(* Logix 5000 AddOnInstructionDefinition export CM1T_CMLDataExchange; software revision 20.00 *)

TYPE CM1T_CMLDriveStatus :
STRUCT
   StatusValue : SINT;   // Indicates status and error type
   StatusValue1 : SINT;   // Additional status values
   In_Position : BOOL;   // Drive is in position and ready to move
   Moving : BOOL;   // Drive is currently moving
   Disabled : BOOL;   // Drive is disabled
   Error : BOOL;   // Drive is in an error state
   HomeAchieved : BOOL;   // Home achieved
END_STRUCT
END_TYPE

TYPE CM1T_CMLAxis :   // CML Axis
STRUCT
   Input : SINT[60];   // Data coming from the CM1-T
   Output : SINT[44];   // Data going to the CM1-T
   us50Counter : DINT;   // Controller 50us counter
   DriveStatus : CM1T_CMLDriveStatus;   // Shows status of the drive
   PositionActual : DINT;   // Actual position of the drive
   TargetActual : DINT;   // 1ms position target
   PositionError : DINT;   // Error between the current drive position and the instantaneous target position
   SpeedActual : DINT;   // Actual speed of the drive
   CurrentActual : INT;   // 0.1% of rated current
   OverloadActual : INT;   // 0.1% of overload torque
   DCVoltage : INT;   // DC voltage bus. 0.1V unit
   AnalogIN : INT;   // Value of 10bit analog input
   DigitalIN : SINT;   // Read the digital inputs
   DigitalOUT : SINT;   // Set the digital outputs
   Temperature : SINT;   // Temperature of the drive
   ErrorCode : SINT;   // Indicates error in Ethernet/IP module
   WriteValue : DINT[5];   // Write value array
   ReadValue : DINT[5];   // Read Value array
   WriteAddr : INT[5];   // Write Address array
   ReadAddr : INT[5];   // Read Address array
   ReadValueAddr : INT[5];   // Address of ReadValue
END_STRUCT
END_TYPE

ADD_ON_INSTRUCTION CM1T_CMLDataExchange   (* revision 1.2, vendor Myostat Motion Control *)
// CM1T CML Data Exchange
VAR_IN_OUT
   DriveInput : AB:ETHERNET_MODULE_SINT_60Bytes:I:0; {required}
   DriveOutput : AB:ETHERNET_MODULE_SINT_44Bytes:O:0; {required}
        .DATA[0]   // Copy outputs to drive
   CM1T_CMLAxis : CM1T_CMLAxis; {required}
        .CONTROLWORD.START   // Controlword.Start Off
        .INPUT   // Copy input from drive
        .OUTPUT[0]   // Write Value1
        .OUTPUT[4]   // Write Value2
        .OUTPUT[8]   // Write Value3
        .OUTPUT[10]   // AccelerationTarget
        .OUTPUT[12]   // Write Value4
        .OUTPUT[14]   // Controlword
        .OUTPUT[16]   // Write Value5
        .OUTPUT[17]   // WriteData
        .OUTPUT[18]   // WriteAddress
        .OUTPUT[20]   // Write Addr1
        .OUTPUT[21]   // Digital OUT
        .OUTPUT[22]   // Write Addr2
        .OUTPUT[24]   // Write Addr3
        .OUTPUT[26]   // Write Addr4
        .OUTPUT[28]   // Write Addr5
        .OUTPUT[30]   // Read Addr1
        .OUTPUT[32]   // Read Addr2
        .OUTPUT[34]   // Read Addr3
        .OUTPUT[36]   // Read Addr4
        .OUTPUT[38]   // Read Addr5
        .DRIVESTATUS.STATUSVALUE   // Status
        .DRIVESTATUS.IN_POSITION   // In Position
        .DRIVESTATUS.MOVING   // Moving
        .DRIVESTATUS.ERROR   // Error
        .POSITIONACTUAL   // Position
        .POSITIONERROR   // Position Error
        .CURRENTACTUAL   // Current
        .DCVOLTAGE   // DC Voltage
        .ANALOGIN   // AnalogIN
        .DIGITALIN   // DigitalIN
        .MODEOFOPERATIONDISPLAY   // Mode Display
        .SPEEDACTUAL   // Speed
        .OVERLOADACTUAL   // Torque
        .TEMPERATURE   // Temperature
        .ERRORCODE   // ErrorCode
END_VAR

ROUTINE Logic   (* ladder *)
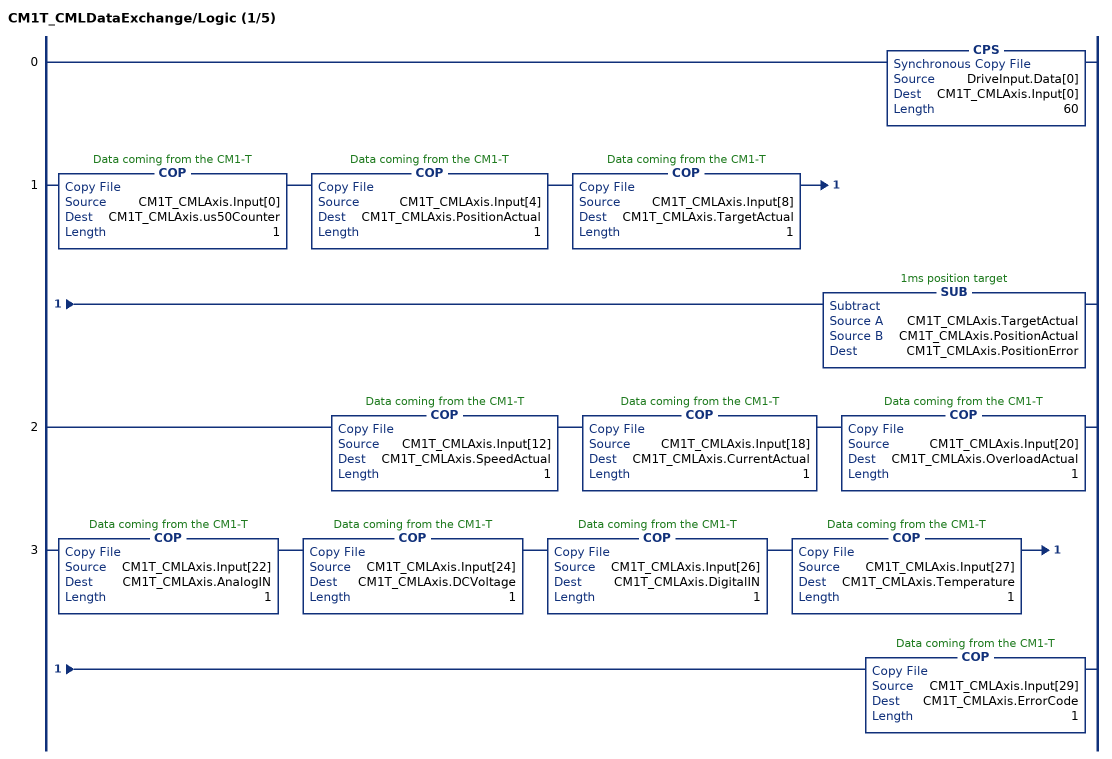
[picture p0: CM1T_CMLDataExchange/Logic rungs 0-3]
   0: CPS(DriveInput.Data[0],CM1T_CMLAxis.Input[0],60);
   1: COP(CM1T_CMLAxis.Input[0],CM1T_CMLAxis.us50Counter,1)COP(CM1T_CMLAxis.Input[4],CM1T_CMLAxis.PositionActual,1)COP(CM1T_CMLAxis.Input[8],CM1T_CMLAxis.TargetActual,1)SUB(CM1T_CMLAxis.TargetActual,CM1T_CMLAxis.PositionActual,CM1T_CMLAxis.PositionError);
   2: COP(CM1T_CMLAxis.Input[12],CM1T_CMLAxis.SpeedActual,1)COP(CM1T_CMLAxis.Input[18],CM1T_CMLAxis.CurrentActual,1)COP(CM1T_CMLAxis.Input[20],CM1T_CMLAxis.OverloadActual,1);
   3: COP(CM1T_CMLAxis.Input[22],CM1T_CMLAxis.AnalogIN,1)COP(CM1T_CMLAxis.Input[24],CM1T_CMLAxis.DCVoltage,1)COP(CM1T_CMLAxis.Input[26],CM1T_CMLAxis.DigitalIN,1)COP(CM1T_CMLAxis.Input[27],CM1T_CMLAxis.Temperature,1)COP(CM1T_CMLAxis.Input[29],CM1T_CMLAxis.ErrorCode,1);
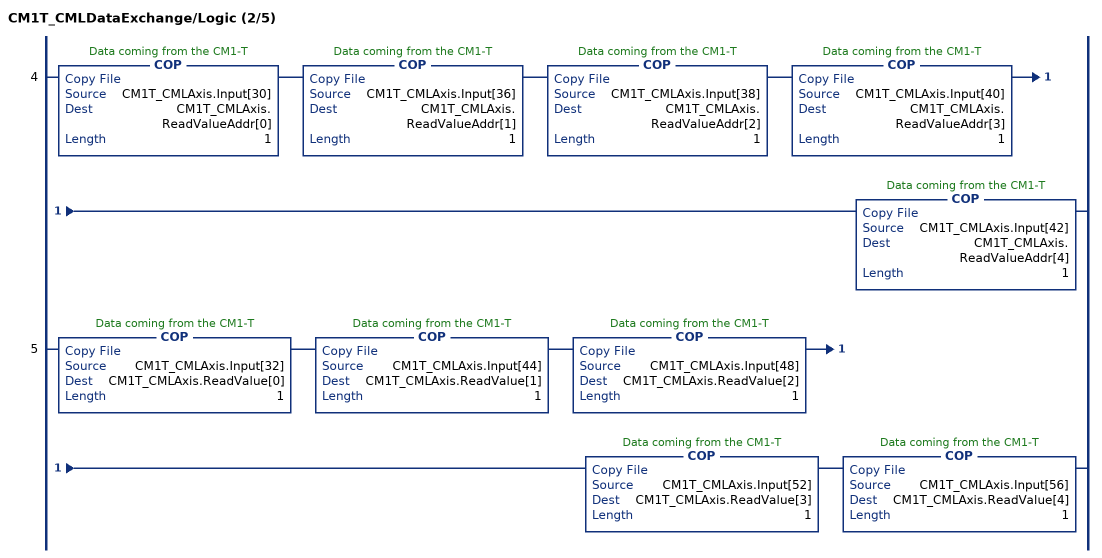
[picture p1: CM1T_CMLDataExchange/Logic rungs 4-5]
   4: COP(CM1T_CMLAxis.Input[30],CM1T_CMLAxis.ReadValueAddr[0],1)COP(CM1T_CMLAxis.Input[36],CM1T_CMLAxis.ReadValueAddr[1],1)COP(CM1T_CMLAxis.Input[38],CM1T_CMLAxis.ReadValueAddr[2],1)COP(CM1T_CMLAxis.Input[40],CM1T_CMLAxis.ReadValueAddr[3],1)COP(CM1T_CMLAxis.Input[42],CM1T_CMLAxis.ReadValueAddr[4],1);
   5: COP(CM1T_CMLAxis.Input[32],CM1T_CMLAxis.ReadValue[0],1)COP(CM1T_CMLAxis.Input[44],CM1T_CMLAxis.ReadValue[1],1)COP(CM1T_CMLAxis.Input[48],CM1T_CMLAxis.ReadValue[2],1)COP(CM1T_CMLAxis.Input[52],CM1T_CMLAxis.ReadValue[3],1)COP(CM1T_CMLAxis.Input[56],CM1T_CMLAxis.ReadValue[4],1);
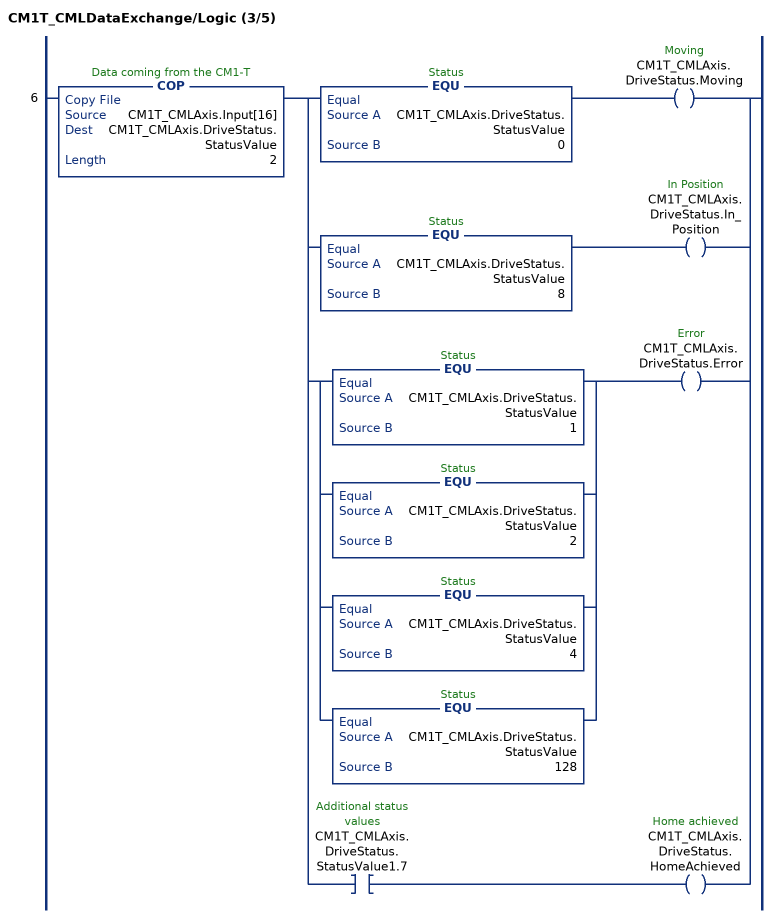
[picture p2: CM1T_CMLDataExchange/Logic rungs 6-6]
   6: COP(CM1T_CMLAxis.Input[16],CM1T_CMLAxis.DriveStatus.StatusValue,2)[EQU(CM1T_CMLAxis.DriveStatus.StatusValue,0) OTE(CM1T_CMLAxis.DriveStatus.Moving) ,EQU(CM1T_CMLAxis.DriveStatus.StatusValue,8) OTE(CM1T_CMLAxis.DriveStatus.In_Position) ,[EQU(CM1T_CMLAxis.DriveStatus.StatusValue,1) ,EQU(CM1T_CMLAxis.DriveStatus.StatusValue,2) ,EQU(CM1T_CMLAxis.DriveStatus.StatusValue,4) ,EQU(CM1T_CMLAxis.DriveStatus.StatusValue,128) ] OTE(CM1T_CMLAxis.DriveStatus.Error) ,XIC(CM1T_CMLAxis.DriveStatus.StatusValue1.7) OTE(CM1T_CMLAxis.DriveStatus.HomeAchieved) ];
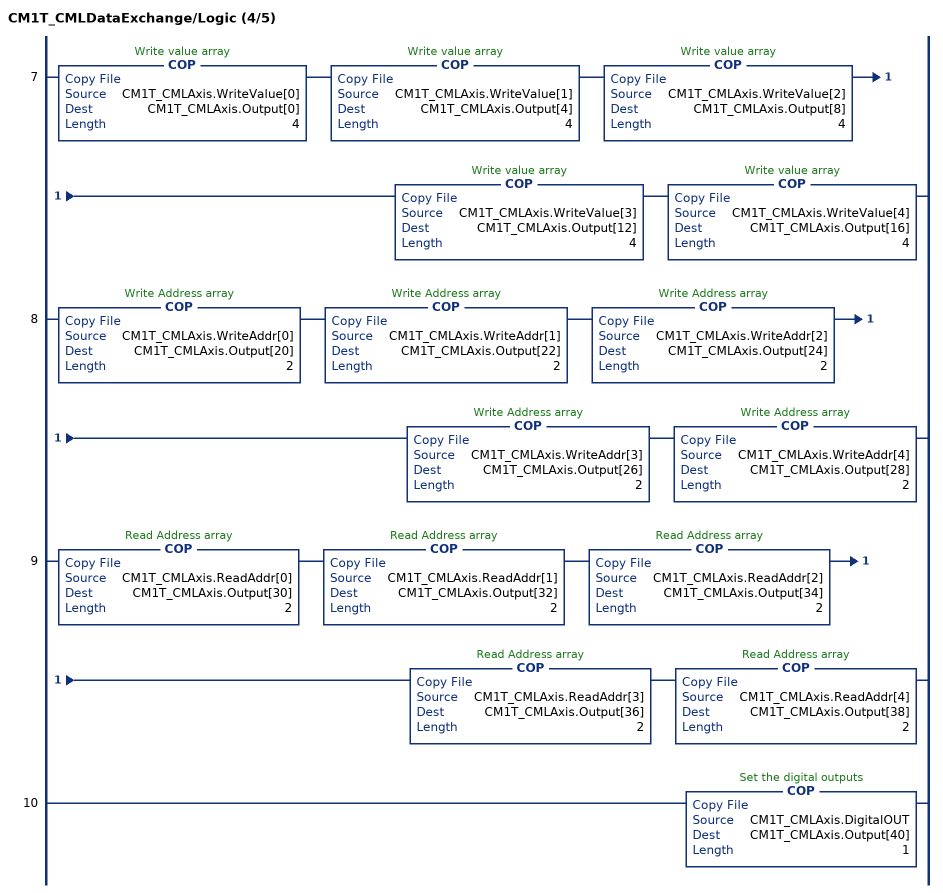
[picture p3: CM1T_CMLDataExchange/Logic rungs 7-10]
   7: COP(CM1T_CMLAxis.WriteValue[0],CM1T_CMLAxis.Output[0],4)COP(CM1T_CMLAxis.WriteValue[1],CM1T_CMLAxis.Output[4],4)COP(CM1T_CMLAxis.WriteValue[2],CM1T_CMLAxis.Output[8],4)COP(CM1T_CMLAxis.WriteValue[3],CM1T_CMLAxis.Output[12],4)COP(CM1T_CMLAxis.WriteValue[4],CM1T_CMLAxis.Output[16],4);
   8: COP(CM1T_CMLAxis.WriteAddr[0],CM1T_CMLAxis.Output[20],2)COP(CM1T_CMLAxis.WriteAddr[1],CM1T_CMLAxis.Output[22],2)COP(CM1T_CMLAxis.WriteAddr[2],CM1T_CMLAxis.Output[24],2)COP(CM1T_CMLAxis.WriteAddr[3],CM1T_CMLAxis.Output[26],2)COP(CM1T_CMLAxis.WriteAddr[4],CM1T_CMLAxis.Output[28],2);
   9: COP(CM1T_CMLAxis.ReadAddr[0],CM1T_CMLAxis.Output[30],2)COP(CM1T_CMLAxis.ReadAddr[1],CM1T_CMLAxis.Output[32],2)COP(CM1T_CMLAxis.ReadAddr[2],CM1T_CMLAxis.Output[34],2)COP(CM1T_CMLAxis.ReadAddr[3],CM1T_CMLAxis.Output[36],2)COP(CM1T_CMLAxis.ReadAddr[4],CM1T_CMLAxis.Output[38],2);
   10: COP(CM1T_CMLAxis.DigitalOUT,CM1T_CMLAxis.Output[40],1);
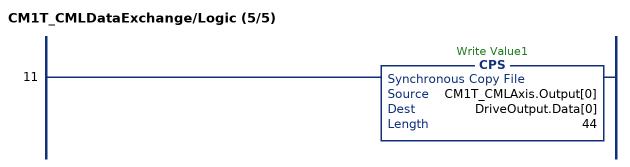
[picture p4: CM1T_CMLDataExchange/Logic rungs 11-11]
   11: CPS(CM1T_CMLAxis.Output[0],DriveOutput.Data[0],44);
END_ROUTINE
END_ADD_ON_INSTRUCTION
